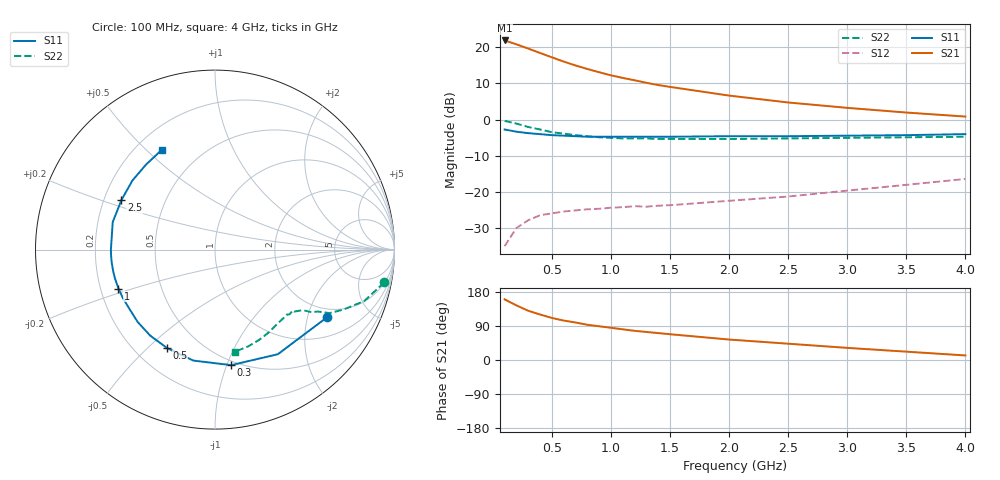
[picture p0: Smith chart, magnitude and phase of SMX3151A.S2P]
! HSMX3151 Common Emitter
! Vce=10V Ic=5ma
# ghz s ma r 50
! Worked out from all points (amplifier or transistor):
!   20 points, 100 MHz to 4 GHz, reference 50 ohm
!   highest |S21| = 21.8 dB at 100 MHz (marker M1)
!   |S21| within 3 dB of that: start of sweep to 362.8 MHz
!   unconditionally stable (mu >= 1): 1.335 GHz to 3.854 GHz
!   at 400 MHz: K = 0.36, MSG = 22.4 dB, |S12| = -26.4 dB
!   at 1.1 GHz: K = 0.86, MSG = 17.8 dB, |S12| = -24.2 dB
!   at 4 GHz: K = 0.96, MSG = 8.6 dB, |S12| = -16.4 dB
!   S11 on the Smith chart (normalised r, x): 100 MHz: 1.66, -2.67; 300 MHz: 0.47, -1.04; 500 MHz: 0.33, -0.58; 1 GHz: 0.28, -0.18; 2.5 GHz: 0.27, +0.23; 4 GHz: 0.30, +0.56
0.1  0.73 -31.0  12.31 160.0  0.018 71.0  0.96 -11.0
0.2  0.68 -59.0  10.89 144.0  0.032 62.0  0.88 -19.0
0.3  0.65 -82.0  9.52 130.0  0.041 53.0  0.79 -25.0
0.4  0.63 -101.0  8.27 120.0  0.048 45.0  0.73 -29.0
0.5  0.61 -116.0  7.21 111.0  0.051 41.0  0.67 -31.0
0.6  0.6 -127.0  6.3 104.0  0.054 40.0  0.64 -33.0
0.7  0.59 -137.0  5.57 99.0  0.056 38.0  0.61 -34.0
0.8  0.58 -145.0  4.98 93.0  0.058 38.0  0.59 -35.0
0.9  0.58 -152.0  4.49 89.0  0.059 37.0  0.57 -37.0
1  0.58 -158.0  4.07 85.0  0.061 37.0  0.56 -38.0
1.1  0.58 -164.0  3.75 81.0  0.062 38.0  0.55 -38.0
1.2  0.58 -168.0  3.48 77.0  0.064 38.0  0.55 -40.0
1.3  0.58 -173.0  3.21 74.0  0.063 38.0  0.55 -41.0
1.4  0.58 -177.0  2.99 71.0  0.065 40.0  0.54 -42.0
1.5  0.58 180.0  2.82 68.0  0.066 41.0  0.54 -44.0
2  0.59 165.0  2.14 54.0  0.076 47.0  0.54 -50.0
2.5  0.59 152.0  1.72 43.0  0.087 53.0  0.55 -57.0
3  0.6 140.0  1.45 32.0  0.105 56.0  0.56 -64.0
3.5  0.61 129.0  1.25 22.0  0.126 57.0  0.57 -71.0
4  0.63 118.0  1.1 12.0  0.152 56.0  0.58 -79.0
